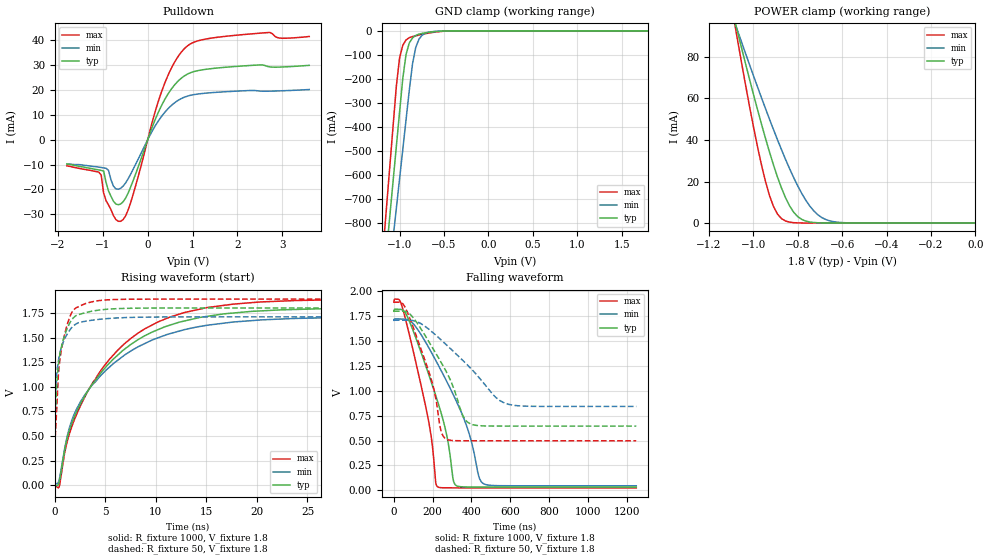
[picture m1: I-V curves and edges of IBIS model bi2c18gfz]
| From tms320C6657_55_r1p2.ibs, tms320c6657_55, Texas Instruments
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| iclkrx10g_1.ibs  [08Jul11 revision 1.2]
|   Model Cell bi2c18gfz
| bi2c18gfz [15July11 revision 1.0]
[Model]   bi2c18gfz
Model_type   I/O_open_drain
Polarity   Non-Inverting
Enable   Active-Low
Vinl =  0.54
Vinh =  1.26
Cref =  400pF
Vref =  1.8V
Rref= 800
Vmeas =  0.9
C_comp   3.56717p   3.42092p   3.71374p
[Model Spec]
Vinl   0.54   0.513   0.567
Vinh   1.26   1.197   1.323
D_overshoot_high 2.34 2.34 2.34
D_overshoot_low -0.3 -0.3 -0.3
D_overshoot_time 1.00E-09 1.00E-09 1.00E-09
S_overshoot_high 1.98 1.98 1.98
S_overshoot_low 0 0 0
[Temperature Range]   25   105   -40
[Voltage Range]   1.8   1.71   1.89
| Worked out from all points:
|   slope of the pulldown table from 0 to 0.27 V, typ, clamps not added: 21.9 ohm
|   GND clamp passes 1 mA (typ) near -0.50 V on its own axis
|   POWER clamp passes 1 mA (typ) near -0.76 V on its own axis
|   rising waveform, R_fixture 1000, V_fixture 1.8: 20-80 % time 6.73ns typ, 6.76ns min, 6.74ns max; typ from 0.033 V to 1.8 V
|   rising waveform, R_fixture 50, V_fixture 1.8: 20-80 % time 1.03ns typ, 1.12ns min, 990ps max; typ from 0.646 V to 1.8 V
|   falling waveform, R_fixture 1000, V_fixture 1.8: 20-80 % time 158ns typ, 217ns min, 116ns max; typ from 1.8 V to 0.033 V
|   falling waveform, R_fixture 50, V_fixture 1.8: 20-80 % time 176ns typ, 258ns min, 123ns max; typ from 1.8 V to 0.646 V
[POWER_clamp]
|   voltage   I(typ)   I(min)   I(max)
-1.8V     430.2mA    330.3mA    582.3mA
-1.091V   100.8mA    98.89mA    100.6mA
-1.073V   92.89mA    93.28mA    89.33mA
-1V       62.31mA    71.21mA    46.79mA
-945.5mV  40.95mA    55.26mA    20.21mA
-909.1mV  27.99mA    45.03mA    7.979mA
-854.5mV  12.11mA    30.6mA     964.9uA
-818.2mV  5.226mA    21.88mA    176.2uA
-781.8mV  1.754mA    14.25mA    30.67uA
-727.3mV  256.4uA    5.814mA    2.178uA
-672.7mV  33.05uA    1.657mA    160.6nA
0V        654.8pA    4.606nA    186.7pA
[Pulldown]
|   voltage   I(typ)   I(min)   I(max)
-1.8V     -9.7mA     -9.8mA     -10.5mA
-1.091V   -12.15mA   -11.02mA   -13.02mA
-1.036V   -12.34mA   -11.16mA   -14.18mA
-981.8mV  -12.56mA   -11.31mA   -21.45mA
-927.3mV  -17.18mA   -11.5mA    -24.54mA
-763.6mV  -24.74mA   -18.66mA   -30.52mA
-600mV    -25.85mA   -19.5mA    -32.83mA
-381.8mV  -19.15mA   -13.93mA   -25.44mA
327.3mV   14.43mA    9.839mA    20.24mA
818.2mV   25.72mA    17.14mA    36.7mA
1.909V    29.44mA    19.51mA    41.98mA
3.6V      29.97mA    20.23mA    41.58mA
[GND_clamp]
|   voltage   I(typ)   I(min)   I(max)
-1.8V     -3.512A    -3.334A    -3.739A
-1.182V   -1.057A    -1.233A    -894.8mA
-1.145V   -913.2mA   -1.109A    -728mA
-1.109V   -769.2mA   -986mA     -561.4mA
-1.073V   -625.4mA   -862.8mA   -395mA
-1.036V   -481.7mA   -739.7mA   -230.4mA
-1V       -338.1mA   -616.6mA   -112.2mA
-927.3mV  -98.58mA   -370.9mA   -38.06mA
-890.9mV  -50.59mA   -248.2mA   -28.47mA
-818.2mV  -19.16mA   -69.23mA   -20.94mA
-672.7mV  -6.283mA   -5.801mA   -9.388mA
1.8V      654.8pA    4.899nA    129.2pA
[Ramp]
| variable   typ   min   max
dV/dt_f   0.69297/0.1762747u   0.520302/0.25845479u   0.83604/0.1229281u
dV/dt_r 38.456058m/0.30108116n 29.167842m/0.30956106n 49.310946m/0.29737873n
R_load = 50
[Rising Waveform]
R_fixture = 1000
V_fixture = 1.8
V_fixture_min = 1.71
V_fixture_max = 1.89
|   time   V(typ)   V(min)   V(max)
0s        33.34mV    45.84mV    24.81mV
430.1ps   29.69mV    53.21mV    -17.54mV
961.6ps   350.4mV    364.8mV    319mV
1.389ns   538.1mV    562mV      502.2mV
2.562ns   832.1mV    851.1mV    812.3mV
5.114ns   1.209V     1.173V     1.241V
8.216ns   1.477V     1.405V     1.544V
15.09ns   1.715V     1.625V     1.805V
26.77ns   1.792V     1.701V     1.883V
1.25us    1.8V       1.71V      1.89V
[Rising Waveform]
R_fixture = 50
V_fixture = 1.8
V_fixture_min = 1.71
V_fixture_max = 1.89
|   time   V(typ)   V(min)   V(max)
0s        646.4mV    843.2mV    497.9mV
87.69ps   813.9mV    964.6mV    559.7mV
266ps     1.119V     1.203V     961.9mV
374.4ps   1.235V     1.277V     1.149V
514.6ps   1.336V     1.347V     1.285V
1.055ns   1.546V     1.503V     1.565V
1.655ns   1.677V     1.599V     1.749V
3.458ns   1.763V     1.673V     1.857V
7.107ns   1.797V     1.703V     1.889V
1.25us    1.8V       1.71V      1.89V
[Falling Waveform]
R_fixture = 1000
V_fixture = 1.8
V_fixture_min = 1.71
V_fixture_max = 1.89
|   time   V(typ)   V(min)   V(max)
0s        1.8V       1.71V      1.891V
35.94ns   1.819V     1.723V     1.884V
89.16ns   1.655V     1.695V     1.487V
175.4ns   1.188V     1.449V     736.2mV
213.8ns   964.6mV    1.314V     100.9mV
225.1ns   894.9mV    1.272V     35.58mV
268.7ns   587.7mV    1.109V     25.47mV
313.1ns   64.33mV    934mV      25.19mV
457.6ns   33.49mV    72.49mV    25.17mV
1.25us    33.48mV    46.2mV     25.17mV
[Falling Waveform]
R_fixture = 50
V_fixture = 1.8
V_fixture_min = 1.71
V_fixture_max = 1.89
|   time   V(typ)   V(min)   V(max)
0s        1.8V       1.71V      1.891V
47.63ns   1.801V     1.711V     1.872V
90.43ns   1.756V     1.708V     1.687V
192.6ns   1.454V     1.6V       1.118V
241.2ns   1.294V     1.516V     610.1mV
266.9ns   1.205V     1.47V      518.8mV
356.2ns   748mV      1.305V     498.3mV
406.4ns   660.2mV    1.205V     498.2mV
593.1ns   646.1mV    864mV      498.2mV
1.25us    646.1mV    843.5mV    498.2mV
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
